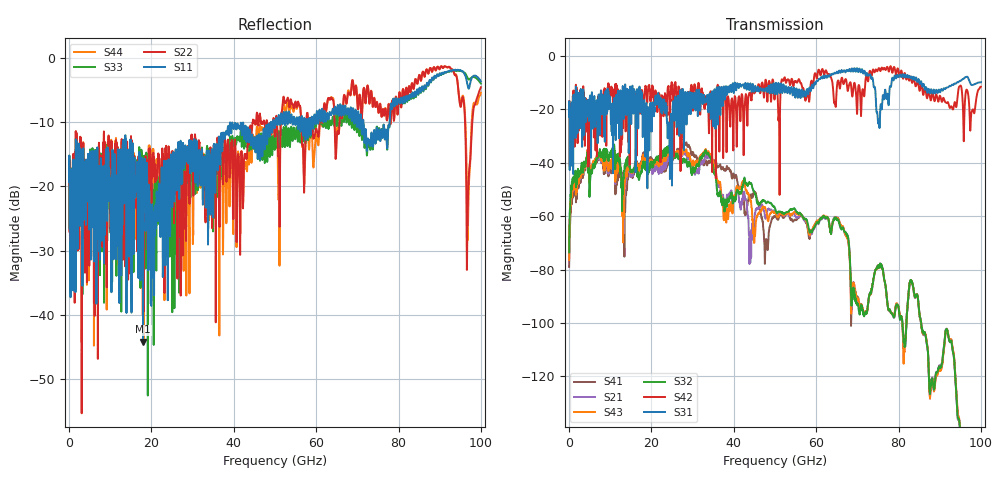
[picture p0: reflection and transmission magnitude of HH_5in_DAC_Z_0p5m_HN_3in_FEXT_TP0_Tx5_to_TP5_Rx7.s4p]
# GHz S RI R 45
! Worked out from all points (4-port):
!   4000 points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, 25 MHz to 100 GHz, reference 45 ohm
!   strongest paths, dB at 25 MHz, 25.02 GHz, 50.02 GHz, 75.03 GHz, 100 GHz:
!     S31: -22.7, -42.9, -13.2, -24.9, -9.8
!     S42: -22.5, -11.1, -12.9, -5.1, -11.5
!     S32: -73.5, -35.5, -57.1, -78.8, -180.8
!     S43: -76.4, -35.6, -58.6, -78.9, -186.5
!     S21: -76.5, -36.3, -58.5, -78.8, -179.6
!     S41: -79.0, -37.1, -60.0, -78.9, -185.4
!   lowest |S11| = -44.2 dB at 17.98 GHz (marker M1), VSWR 1.01, Z = 45.1 - j0.554 ohm
!   |S11| at or under -10 dB: start of sweep to 48.99 GHz; 49.09 GHz to 49.52 GHz (422.7 MHz wide, 0.857 % of centre); 71.51 GHz to 77.87 GHz (6.365 GHz wide, 8.52 % of centre)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
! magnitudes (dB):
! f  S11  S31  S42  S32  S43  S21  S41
! 25 MHz  -19.3  -22.7  -22.5  -73.5  -76.4  -76.5  -79.0
! 4.375 GHz  -19.7  -20.0  -20.8  -38.4  -38.0  -37.9  -38.6
! 17.98 GHz  -44.2  -27.0  -17.9  -40.4  -37.4  -38.2  -36.6
! 33.45 GHz  -14.5  -15.9  -17.0  -36.6  -36.1  -37.8  -40.4
! 38.7 GHz  -10.9  -11.6  -15.9  -54.8  -59.3  -53.6  -42.1
! 47.88 GHz  -10.5  -12.1  -9.8  -55.1  -58.1  -60.2  -68.6
! 100 GHz  -3.6  -9.8  -11.5  -180.8  -186.5  -179.6  -185.4
